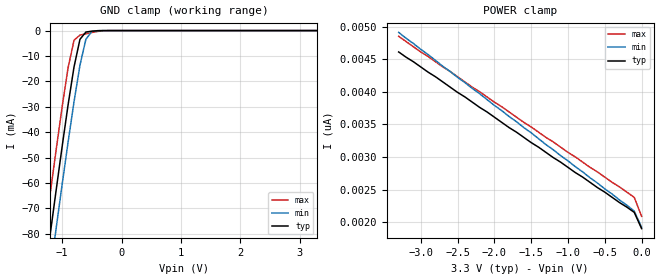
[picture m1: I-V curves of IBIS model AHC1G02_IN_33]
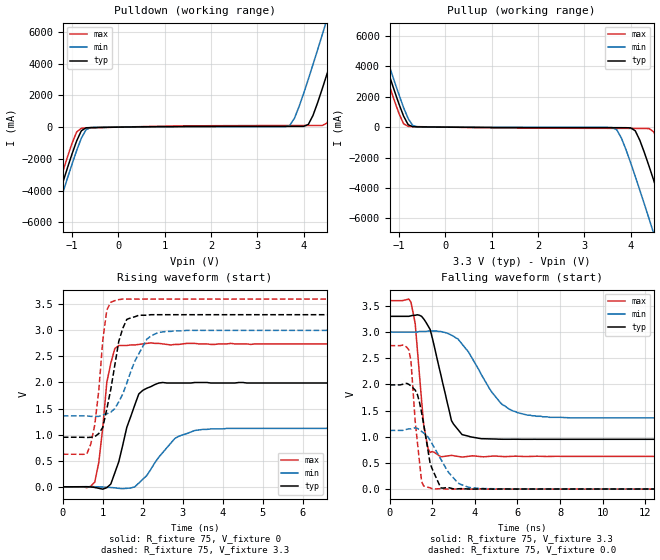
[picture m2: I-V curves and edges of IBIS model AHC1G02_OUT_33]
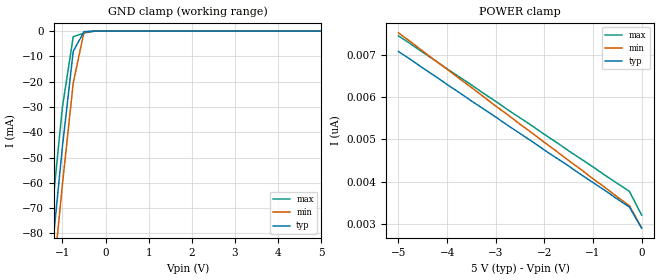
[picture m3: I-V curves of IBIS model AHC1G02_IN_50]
| TEXAS INSTRUMENTS INCORPORATED
| Standard Linear and Logic Group
| IBIS Model of SN74AHC1G02
| SINGLE 2-INPUT POSITIVE-NOR GATE
| SOT 5-pin (DCK) and SOT 5-pin (DBV) Package
[IBIS Ver]   3.2
[Comment Char]  |_char
[File Name]   ahc1g02.ibs
[File Rev]   2.0 J_die
[Date]   May 24, 2000
[Source]   Data created from HSPICE simulations at TI-SLL.
[Notes]   The following is an IBIS list for the AHC1G02.
|   Please contact sllibis@ti.com with questions and
|   comments concerning SLL IBIS models.
[Disclaimer] Property of Texas Instruments Incorporated.  Unauthorized
   reproduction and/or distribution is strictly prohibited.
   This product is protected under copyright law.
   Created 2000, (C) Copyright 2000, Texas Instruments Inc.,
   All Rights Reserved.
   UNLESS THERE IS A SIGNED, WRITTEN AGREEMENT TO THE
   CONTRARY, TEXAS INSTRUMENTS () IS PROVIDING THE IBIS
   MODELS  AND WITHOUT ANY WARRANTY, EXPRESSED OR
   IMPLIED.  TI assumes no liability for:
   1) the accuracy of the IBIS models provided to your
   company;
   2) the proper functioning of these IBIS Models in your
   design or for any resulting applications; or
   3) infringement of patents, copyrights or intellectual
   property rights resulting from your use of these IBIS
   models.
   TI provides IBIS Models as a service to our customers.
   You and your company shall not distribute, sell or give
   these models to anyone else without prior written
   permission from TI.
   TI reserves the right to make changes to our products or
   to discontinue any semiconductor product or service
   without notice, and advises our customers to obtain the
   latest version of relevant information to verify, before
   placing orders, that the information being relied on is
   current.
   Please be aware that your receipt and use of the IBIS
   information provided shall serve as acceptance of these
   terms and conditions.  If you do not accept these terms,
   you should return or destroy the IBIS models and any
   other accompanying information immediately.
|   Component AHC1G02_DCK
[Component]   AHC1G02_DCK
[Manufacturer]  Texas Instruments, Inc.
[Package]
|   typ   min   max
R_pkg   0.020   0.017   0.025
L_pkg   0.998nH   0.881nH   1.069nH
C_pkg   0.146pF   0.118pF   0.205pF
[Pin]   signal_name   model_name   R_pin   L_pin   C_pin
1   A   AHC1G02_IN   0.019   1.069nH   0.162pF
2   B   AHC1G02_IN   0.018   0.881nH   0.121pF
3   GND   GND   0.017   1.031nH   0.205pF
4   Y   AHC1G02_OUT   0.020   0.960nH   0.124pF
5   VCC   POWER   0.025   1.049nH   0.118pF
|   Component AHC1G02_DBV
[Component]   AHC1G02_DBV
[Manufacturer]  Texas Instruments, Inc.
[Package]
|   typ   min   max
R_pkg   0.025   0.021   0.029
L_pkg   1.529nH   1.312nH   1.906nH
C_pkg   0.156pF   0.110pF   0.240pF
[Pin]   signal_name   model_name   R_pin   L_pin   C_pin
1   A   AHC1G02_IN   0.021   1.511nH   0.144pF
2   B   AHC1G02_IN   0.023   1.312nH   0.138pF
3   GND   GND   0.029   1.906nH   0.240pF
4   Y   AHC1G02_OUT   0.026   1.541nH   0.150pF
5   VCC   POWER   0.025   1.374nH   0.110pF
[Model Selector]   AHC1G02_IN
AHC1G02_IN_33   3.3-V Vcc Input Model
AHC1G02_IN_50   5.0-V Vcc Input Model
[Model Selector]   AHC1G02_OUT
AHC1G02_OUT_33   3.3-V Vcc Output Model
AHC1G02_OUT_50   5.0-V Vcc Output Model
| Models and submodels in the file (4): AHC1G02_IN_33 (Input), AHC1G02_OUT_33 (Output), AHC1G02_IN_50 (Input), AHC1G02_OUT_50 (Output)
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|   Model AHC1G02_IN_33
[Model]   AHC1G02_IN_33
Model_type  Input
Polarity   Inverting
Vinl = 0.99
Vinh = 2.31
| variable   typ   min   max
C_comp   1.27pf   0.95pf   1.59pf
[Temperature Range]   25   85   -40
[Voltage Range]   3.3   3.0   3.6
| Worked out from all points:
|   GND clamp passes 1 mA (typ) near -0.61 V on its own axis
[GND Clamp]
|   Voltage   I(typ)   I(min)   I(max)
-3.3V     -460mA     -475mA     -445mA
-1.3V     -97.5mA    -113mA     -81.5mA
-1.2V     -79.9mA    -95mA      -63.9mA
-1.1V     -62.6mA    -77.6mA    -46.7mA
-1V       -45.6mA    -60.5mA    -30mA
-900mV    -29.2mA    -43.9mA    -14.6mA
-800mV    -14.3mA    -28mA      -3.81mA
-700mV    -3.42mA    -13.6mA    -1.78mA
-600mV    -581uA     -3.4mA     -1.25mA
-500mV    -233uA     -353uA     -759uA
-400mV    -58.1uA    -21.9uA    -324uA
3.3V      1.9nA      2.34nA     1.69nA
[POWER Clamp]
|   Voltage   I(typ)   I(min)   I(max)
-3.3V     4.61nA     4.91nA     4.85nA
-3V       4.38nA     4.65nA     4.61nA
-100mV    2.15nA     2.17nA     2.38nA
0V        1.9nA      1.92nA     2.09nA
|   Model AHC1G02_OUT_33
[Model]   AHC1G02_OUT_33
Model_type  Output
Polarity   Inverting
Vmeas = 1.65v
Cref = 15pf
| variable   typ   min   max
C_comp   3.12pf   2.34pf   3.90pf
[Temperature Range]   25   85   -40
[Voltage Range]   3.3   3.0   3.6
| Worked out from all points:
|   slope of the pulldown table from 0 to 0.495 V, typ, clamps not added: 26.1 ohm
|   slope of the pullup table from 0 to 0.495 V, typ, clamps not added: 40.3 ohm
|   rising waveform, R_fixture 75, V_fixture 0: 20-80 % time 449ps typ, 660ps min, 240ps max; typ from 0 V to 1.99 V
|   falling waveform, R_fixture 75, V_fixture 3.3: 20-80 % time 804ps typ, 1.53ns min, 369ps max; typ from 3.3 V to 0.95 V
|   rising waveform, R_fixture 75, V_fixture 3.3: 20-80 % time 336ps typ, 548ps min, 229ps max; typ from 0.95 V to 3.3 V
|   falling waveform, R_fixture 75, V_fixture 0.0: 20-80 % time 551ps typ, 1.02ns min, 349ps max; typ from 1.99 V to 0 V
[Pulldown]
|   Voltage   I(typ)   I(min)   I(max)
-3.3V     -24A       -24.6A     -23.4A
-1.6V     -7.31A     -7.95A     -6.63A
-1.5V     -6.34A     -6.99A     -5.66A
-1V       -1.69A     -2.33A     -1.02A
-800mV    -234mA     -703mA     -70.7mA
-600mV    -28.4mA    -27.3mA    -48.1mA
3.7V      47.1mA     113mA      100mA
4.1V      173mA      3.03A      101mA
4.4V      2.42A      5.83A      105mA
4.8V      6.17A      9.67A      2.68A
5.2V      10A        13.6A      6.5A
6.6V      23.8A      27.4A      20.3A
[Pullup]
|   Voltage   I(typ)   I(min)   I(max)
-3.3V     23.8A      24.4A      23.2A
-1.6V     7.13A      7.74A      6.5A
-1.5V     6.17A      6.78A      5.53A
-1V       1.53A      2.14A      903mA
-800mV    158mA      559mA      49mA
-600mV    19.5mA     16.8mA     33.4mA
3.7V      -35.9mA    -168mA     -78.9mA
4.1V      -236mA     -3.23A     -83.5mA
4.4V      -2.58A     -6.03A     -95.5mA
4.8V      -6.34A     -9.88A     -2.81A
5.2V      -10.2A     -13.8A     -6.63A
6.6V      -24A       -27.6A     -20.4A
[Ramp]
| variable   typ   min   max
dV/dt_r   1.22E+00/4.32E-10   7.05E-01/7.16E-10   1.65E+00/2.29E-10
dV/dt_f   1.43E+00/7.96E-10   9.98E-01/1.52E-09   1.81E+00/3.68E-10
R_load = 75
[Rising Waveform]
R_fixture = 75
V_fixture = 0
|   Time   V(typ)   V(min)   V(max)
0s        0V         0V         0V
800ps     -13mV      1.3mV      91.3mV
900ps     -28.8mV    -850uV     467mV
1.1ns     -16.6mV    -9.28mV    2V
1.4ns     481mV      -30.4mV    2.71V
1.9ns     1.78V      71.4mV     2.73V
2.5ns     2V         658mV      2.74V
2.9ns     1.99V      969mV      2.73V
4.1ns     1.99V      1.12V      2.74V
25ns      1.99V      1.12V      2.74V
[Falling Waveform]
R_fixture = 75
V_fixture = 3.3
V_fixture_min = 3.0
V_fixture_max = 3.6
|   Time   V(typ)   V(min)   V(max)
0s        3.3V       3V         3.6V
1ns       3.31V      3V         3.57V
1.2ns     3.32V      3V         3.16V
1.8ns     3.12V      3.02V      776mV
2.4ns     2.19V      3.01V      616mV
2.9ns     1.31V      2.94V      643mV
3.4ns     1.04V      2.77V      611mV
5.2ns     952mV      1.65V      624mV
6.5ns     950mV      1.41V      622mV
25ns      950mV      1.36V      624mV
[Rising Waveform]
R_fixture = 75
V_fixture = 3.3
V_fixture_min = 3.0
V_fixture_max = 3.6
|   Time   V(typ)   V(min)   V(max)
0s        950mV      1.36V      624mV
700ps     949mV      1.35V      820mV
800ps     962mV      1.35V      1.19V
1ns       1.14V      1.38V      2.81V
1.1ns     1.49V      1.4V       3.39V
1.4ns     2.79V      1.63V      3.59V
1.6ns     3.21V      1.99V      3.6V
2.1ns     3.29V      2.83V      3.6V
2.6ns     3.3V       2.98V      3.6V
25ns      3.3V       3V         3.6V
[Falling Waveform]
R_fixture = 75
V_fixture = 0.0
|   Time   V(typ)   V(min)   V(max)
0s        1.99V      1.12V      2.74V
900ps     2V         1.15V      2.66V
1ns       1.97V      1.15V      2.45V
1.2ns     1.89V      1.17V      1.29V
1.5ns     1.46V      1.1V       141mV
2ns       382mV      859mV      5.91mV
2.4ns     22.1mV     572mV      3.84mV
3.2ns     3.28mV     119mV      1.28mV
3.8ns     -1mV       26.8mV     -1.88mV
25ns      0V         0V         0V
|   Model AHC1G02_IN_50
[Model]   AHC1G02_IN_50
Model_type  Input
Polarity   Inverting
Vinl = 1.5
Vinh = 3.5
| variable   typ   min   max
C_comp   1.27pf   0.95pf   1.59pf
[Temperature Range]   25   85   -40
[Voltage Range]   5.0   4.5   5.5
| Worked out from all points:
|   GND clamp passes 1 mA (typ) near -0.52 V on its own axis
[GND Clamp]
|   Voltage   I(typ)   I(min)   I(max)
-5V       -773mA     -786mA     -758mA
-1.5V     -133mA     -148mA     -117mA
-1.25V    -88.7mA    -104mA     -72.7mA
-1V       -45.6mA    -60.5mA    -30mA
-750mV    -7.99mA    -20.5mA    -2.23mA
-500mV    -233uA     -353uA     -759uA
-250mV    -2.63nA    -182nA     -26.9uA
5V        2.9nA      3.64nA     2.54nA
[POWER Clamp]
|   Voltage   I(typ)   I(min)   I(max)
-5V       7.08nA     7.52nA     7.45nA
-1.5V     4.37nA     4.5nA      4.73nA
-250mV    3.4nA      3.43nA     3.77nA
0V        2.9nA      2.91nA     3.21nA
